PROGRAM MAIN
VAR
	eState: E_RRCS_State := IDLE;							// state of the statemachine, set this value to CHECK_GATEWAY to execute the request -
			 												// see https://infosys.beckhoff.com/english.php?content=../content/1033/tc3_plc_intro/2531621771.html
	fbRRCScom: FB_RRCScom(
				ipAddr_Server:= '192.168.42.59', 			// the IP-Address of the PC which runs the RRCS-Server
				ipPort_Server:=8193)						// the Port of the PC which runs the RRCS-Server
				:= (eTraceLevel := TcEventSeverity.Verbose);
	tonRetry: TON := (pt := T#5S);							// Retry in case of errors
	tonWait: TON := (pt := T#70MS);
	ui: UINT;
	
	{region 'Get States'}
	bExecuteGetState: BOOL := FALSE;						
	fbGetState: FB_GetState(pfbRRCscom := ADR(fbRRCScom));	// functionblock used to get the state of the RRCS-Server
	{endregion}
	
	{region 'Get Alive'}
	bExecuteGetAlive: BOOL := TRUE;
	fbGetAlive: FB_GetAlive(pfbRRCscom := ADR(fbRRCScom));
	{endregion}

	{region 'Is connected to Artist'}
	bExecuteGetConnectedToArtist: BOOL := TRUE;
	fbIsConnectedToArtist: FB_IsConnectedToArtist(pfbRRCscom := ADR(fbRRCScom));
	{endregion}
	
	{region 'Get Logic Sources'}	  
	bExecuteGetAllLogicSources: BOOL;
	fbGetAllLogicSources_V2: FB_GetAllLogicSources_v2(pfbRRCscom := ADR(fbRRCScom));
	tonGetLogicSourceStates: TON;	
	{endregion}

	{region 'Set a Logic Source'} 
	bState: BOOL;	// the required status
	_bState: BOOL;
	fbSetLogicSourceState: FB_SetLogicSourceState(pfbRRCscom := ADR(fbRRCScom));
	{endregion}
END_VAR

CASE eState OF
	CHECK_GATEWAY: 
		tonRetry(IN := FALSE);
		fbGetState(bExecute:= bExecuteGetState);
		bExecuteGetState:= FALSE;
		IF fbGetState.bError THEN
			eState:= ERROR;
		ELSIF NOT fbGetState.bBusy THEN
			IF fbGetState.sGatewayState = 'Working' THEN
					eState := CHECK_ALIVE;
			ELSE
				eState := ERROR;		 
			END_IF
		END_IF

	CHECK_ALIVE:
		fbGetAlive(bExecute:= bExecuteGetAlive);
		bExecuteGetAlive:= FALSE;
		IF fbGetAlive.bError THEN
			eState:= ERROR;
		ELSIF NOT fbGetAlive.bBusy THEN
			IF fbGetAlive.bAlive THEN
					bExecuteGetConnectedToArtist:= TRUE; 
					eState := CHECK_CONN_ARTIST;
			ELSE
				eState := ERROR;		 
			END_IF
		END_IF
	

	CHECK_CONN_ARTIST:
		fbIsConnectedToArtist(bExecute:= bExecuteGetConnectedToArtist);
		bExecuteGetConnectedToArtist:= FALSE;
		IF fbIsConnectedToArtist.bError THEN
			eState:= ERROR;
		ELSIF NOT fbIsConnectedToArtist.bBusy THEN
			IF fbIsConnectedToArtist.bIsConnected THEN
					eState := GET_SOURCES;
			ELSE
				eState := ERROR;		 
			END_IF
		END_IF

	GET_SOURCES:
		IF bState <> _bState THEN
			_bState := bState;
			eState := SET_SOURCE;
		ELSE
			tonGetLogicSourceStates(in := TRUE, pt:= T#50MS);
			IF tonGetLogicSourceStates.Q THEN
				tonGetLogicSourceStates(In := FALSE);
				bExecuteGetAllLogicSources := TRUE;
			END_IF	
			fbGetAllLogicSources_V2(bExecute:= bExecuteGetAllLogicSources); 
			bExecuteGetAllLogicSources := FALSE;
			IF fbGetAllLogicSources_V2.bError THEN
				fbGetAllLogicSources_V2(bExecute:= FALSE);
				eState:= ERROR;
			ELSIF NOT fbGetAllLogicSources_V2.bBusy AND bExecuteGetAllLogicSources THEN
				fbGetAllLogicSources_V2(bExecute:= FALSE);
				IF fbGetAllLogicSources_V2.eRRCS_ErrorCode <> E_RRCS_ErrorCodes.Success THEN
					eState:= ERROR;
				END_IF	
			END_IF 
		END_IF	

	SET_SOURCE:
		FOR ui := 0 TO PL_RRCS.nMaxLogicSources - 1 DO
			IF fbGetAllLogicSources_V2.aLogicSources[ui].sLabel_8Char = 'Mute A' THEN 
				EXIT;
			END_IF	
	  	END_FOR
		IF ui < PL_RRCS.nMaxLogicSources THEN // Preset found ....
			fbSetLogicSourceState(bExecute := TRUE, bState := bState, 
				nObjectID := fbGetAllLogicSources_V2.aLogicSources[ui].nObjectID,
				aLogicSources := fbGetAllLogicSources_V2.aLogicSources);
				IF fbSetLogicSourceState.bError THEN
					fbSetLogicSourceState(bExecute := FALSE, aLogicSources := fbGetAllLogicSources_V2.aLogicSources);
					eState:= ERROR;
				ELSIF NOT fbSetLogicSourceState.bBusy THEN
					fbSetLogicSourceState(bExecute := FALSE, aLogicSources := fbGetAllLogicSources_V2.aLogicSources);
					eState := WAIT;
				END_IF 
		END_IF
	
	WAIT: 
		tonWAIT(In := NOT tonWAIT.Q);
		IF tonWAIT.Q THEN
			tonWAIT(In := FALSE);
			eState := GET_SOURCES;
		END_IF

	ERROR:
		fbGetState(bExecute:= FALSE);
		tonRetry(In:= NOT tonRetry.Q);
		IF tonRetry.Q THEN
			bExecuteGetState:= TRUE;
			eState:= CHECK_GATEWAY;	
		END_IF

END_CASE

IF NOT tonRetry.Q THEN
	eState := SEL(fbRRCScom.eCommState = E_CommState.ERROR, eState, ERROR);
END_IF

END_PROGRAM
